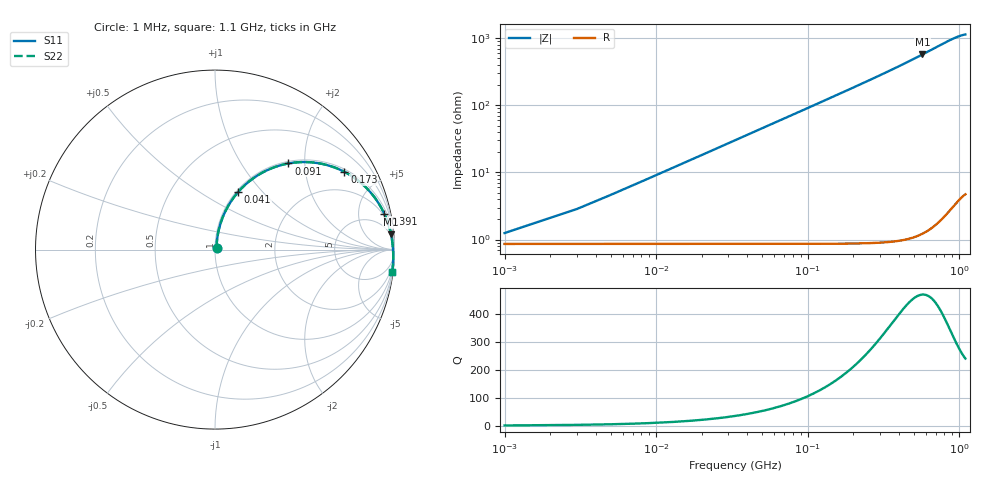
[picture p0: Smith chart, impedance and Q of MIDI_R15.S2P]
! Coilcraft 1812SMS-R15 Spring Air Core Inductor
! 14 FEBRUARY 2008
# MHZ S MA R 50
!Freq  MagS11  AngS11  MagS21  AngS21  MagS12  AngS12  MagS22  AngS22
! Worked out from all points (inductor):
!   551 points, 1 MHz to 1.1 GHz, reference 50 ohm
!   read as one part in series: L = 144 nH near 5 MHz
!   highest Q = 469 at 573 MHz (marker M1), where L = 159 nH
!   S11 on the Smith chart (normalised r, x): 1 MHz: 1.02, +0.02; 41 MHz: 1.02, +0.74; 91 MHz: 1.04, +1.66; 173 MHz: 1.10, +3.27; 391 MHz: 1.64, +9.32; 1.1 GHz: 1, -16
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1  0.01233 45.7  0.9914 -0.5  0.9914 -0.5  0.01234 45.8
3  0.02805 70.8  0.9911 -1.6  0.9911 -1.6  0.02806 70.8
7  0.06285 78.6  0.9895 -3.6  0.9895 -3.6  0.06286 78.6
9  0.08041 79.3  0.9883 -4.7  0.9883 -4.7  0.08043 79.3
11  0.09794 79.3  0.9867 -5.7  0.9867 -5.7  0.09797 79.3
15  0.1328 78.6  0.9827 -7.7  0.9827 -7.7  0.1328 78.6
19  0.1672 77.4  0.9775 -9.8  0.9775 -9.8  0.1672 77.4
25  0.2177 75.0  0.9677 -12.8  0.9677 -12.8  0.2177 75.0
41  0.3435 68.2  0.9312 -20.4  0.9312 -20.4  0.3436 68.2
63  0.4901 59.3  0.8642 -29.9  0.8642 -29.9  0.4903 59.3
91  0.631 49.5  0.7692 -39.9  0.7692 -39.9  0.6311 49.5
131  0.7613 38.9  0.6428 -50.6  0.6428 -50.6  0.7615 38.9
173  0.8414 31.0  0.5357 -58.7  0.5357 -58.7  0.8416 31.0
185  0.8575 29.1  0.5098 -60.6  0.5098 -60.6  0.8578 29.1
261  0.9217 20.5  0.3842 -69.3  0.3842 -69.3  0.922 20.5
369  0.96 13.0  0.277 -76.8  0.277 -76.8  0.9602 13.0
391  0.9645 11.9  0.2613 -78.0  0.2613 -78.0  0.9647 11.9
551  0.983 5.7  0.1809 -84.2  0.1809 -84.2  0.9832 5.7
573  0.9844 5.0  0.1731 -84.9  0.1731 -84.9  0.9846 5.0
735  0.9911 0.7  0.1295 -89.1  0.1295 -89.1  0.9913 0.7
917  0.9944 -3.3  0.1007 -93.1  0.1007 -93.1  0.9946 -3.3
1100  0.9955 -7.1  0.0875 -96.9  0.0875 -96.9  0.9957 -7.1
